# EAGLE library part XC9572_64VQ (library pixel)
xc9536_pc44 XC9500 In-System Programmable CPLD Family Auto generated by make-symbol-device-package-bsdl.ulp Rev. 34 Source: xc9536_vq44.bsd
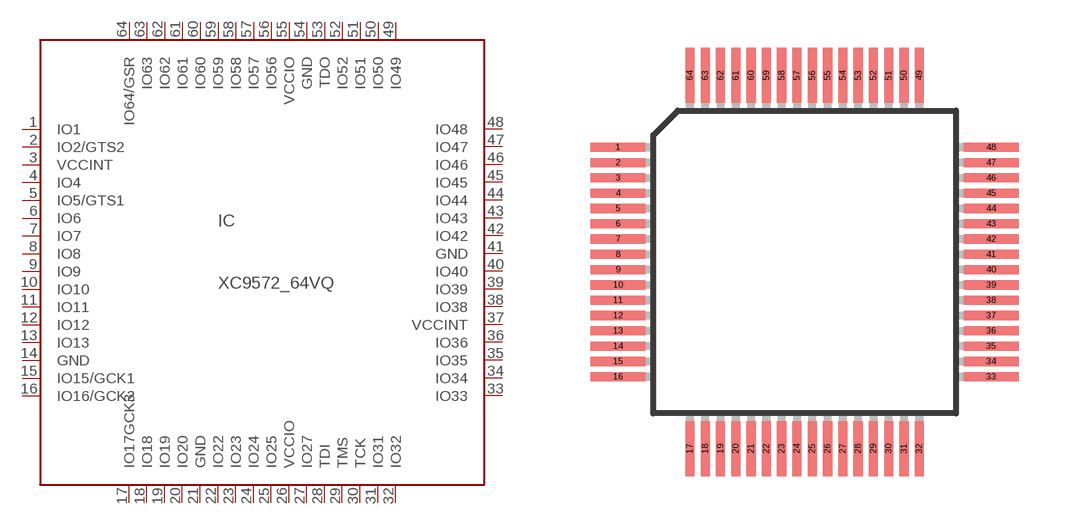
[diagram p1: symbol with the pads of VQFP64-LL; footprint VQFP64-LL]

Designator prefix IC

## XC9572_64VQ (MPN: XC9536-15VQG44C; OC_FARNELL: 1193227; OC_NEWARK: 98K3377)  [VQFP64-LL]
1  IO1
2  IO2/GTS2
3  VCCINT
4  IO4  pwr
5  IO5/GTS1
6  IO6
7  IO7
8  IO8
9  IO9  in
10  IO10  in
11  IO11  in
12  IO12
13  IO13
14  GND
15  IO15/GCK1
16  IO16/GCK2
17  IO17GCK3
18  IO18
19  IO19
20  IO20  pwr
21  GND
22  IO22  pwr
23  IO23
24  IO24
25  IO25
26  VCCIO
27  IO27
28  TDI
29  TMS
30  TCK
31  IO31
32  IO32
33  IO33
34  IO34
35  IO35
36  IO36
37  VCCINT
38  IO38
39  IO39  out
40  IO40  pwr
41  GND  pwr
42  IO42
43  IO43
44  IO44
45  IO45
46  IO46
47  IO47
48  IO48
49  IO49
50  IO50
51  IO51
52  IO52
53  TDO
54  GND
55  VCCIO  in
56  IO56
57  IO57
58  IO58
59  IO59
60  IO60
61  IO61
62  IO62
63  IO63
64  IO64/GSR

## Footprint VQFP64-LL (pad centres in mm)
64-lead VQVP Source. http://www.atmel.com/dyn/resources/prod_documents/doc4136.pdf
smd 1.8 x 0.3: 1 -6.1,3.75; 2 -6.1,3.25; 3 -6.1,2.75; 4 -6.1,2.25; 5 -6.1,1.75; 6 -6.1,1.25; 7 -6.1,0.75; 8 -6.1,0.25; 9 -6.1,-0.25; 10 -6.1,-0.75; 11 -6.1,-1.25; 12 -6.1,-1.75; 13 -6.1,-2.25; 14 -6.1,-2.75; 15 -6.1,-3.25; 16 -6.1,-3.75; 33 6.1,-3.75; 34 6.1,-3.25; 35 6.1,-2.75; 36 6.1,-2.25; 37 6.1,-1.75; 38 6.1,-1.25; 39 6.1,-0.75; 40 6.1,-0.25; 41 6.1,0.25; 42 6.1,0.75; 43 6.1,1.25; 44 6.1,1.75; 45 6.1,2.25; 46 6.1,2.75; 47 6.1,3.25; 48 6.1,3.75
smd 0.3 x 1.8: 17 -3.75,-6.1; 18 -3.25,-6.1; 19 -2.75,-6.1; 20 -2.25,-6.1; 21 -1.75,-6.1; 22 -1.25,-6.1; 23 -0.75,-6.1; 24 -0.25,-6.1; 25 0.25,-6.1; 26 0.75,-6.1; 27 1.25,-6.1; 28 1.75,-6.1; 29 2.25,-6.1; 30 2.75,-6.1; 31 3.25,-6.1; 32 3.75,-6.1; 49 3.75,6.1; 50 3.25,6.1; 51 2.75,6.1; 52 2.25,6.1; 53 1.75,6.1; 54 1.25,6.1; 55 0.75,6.1; 56 0.25,6.1; 57 -0.25,6.1; 58 -0.75,6.1; 59 -1.25,6.1; 60 -1.75,6.1; 61 -2.25,6.1; 62 -2.75,6.1; 63 -3.25,6.1; 64 -3.75,6.1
